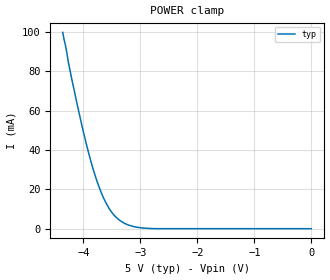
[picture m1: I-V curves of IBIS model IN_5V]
| TEXAS INSTRUMENTS INCORPORATED
| Dual Channel High Speed ESD Protection Device
| Marketing part#   Voltage Range   Package-type   #pins/pkg drawing
| TPD2E1B06DRLR   5.5   SOT   6 / DRL
[IBIS Ver]   4.0
[File name]   tpd2e1b06.ibs
[File Rev]   1.0
[Date]   18-JUL-2013
[Source]
| Texas Instruments Incorporated
| Webench Design Center
| 12500 TI Blvd
| Dallas, TX 75243
| e-mail: elab_scm_ibis@list.ti.com
[Notes]   Revision History:
| Rev 1.0: 18-JUL-2013
| - Initial version of the model
| - Model generated from measurements on Keithley 2420
[Disclaimer]
| This model is designed as an aid for customers of Texas Instruments.
| TI and its licensors and suppliers make no warranties, either expressed
| or implied, with respect to this  model, including the warranties of
| merchantability or fitness for a particular purpose. The model is
| provided solely on an "as is" basis. The entire risk as to its quality
| and performance is with the customer.
[Copyright]
(C) Copyright 2013 Texas Instruments Incorporated. All rights reserved.
|   TPD2E1B06DRL
[Component]   TPD2E1B06DRL
[Manufacturer]   Texas Instruments, Inc.
[Package]   |6 pin DRL SOT package
|   typ   min   max
R_pkg   0.00998   NA   NA
L_pkg   0.60587n   NA   NA
C_pkg   0.18890p   NA   NA
[Pin]   signal_name   model_name   R_pin   L_pin   C_pin
1   IOA1   IN_5V   0.03787   0.61375n   0.10884p
2   IOB1   IN_5V   0.00623   0.52312n   0.18891p
3   NC   NC   0.00998   0.81276n   0.26643p
4   IOB2   GND   0.03772   0.60587n   0.10852p
5   IOA2   GND   0.00623   0.52312n   0.18890p
6   NC   NC   0.00998   0.81270n   0.26639p
| Models and submodels in the file (1): IN_5V (Input)
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|   Model IN_5V
[Model]   IN_5V
Model_type   Input
Vinl = 0
Vinh = 0
|   typ   min   max
C_comp   0.1p   0.1p   0.1p
[Voltage Range]   5   NA   NA
[Temperature Range]   27   NA   NA
[Power Clamp Reference]   5   NA   NA
[GND Clamp Reference]   0   NA   NA
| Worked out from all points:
|   POWER clamp passes 1 mA (typ) near -3.11 V on its own axis
[GND Clamp]
|   Voltage   I(typ)   I(min)   I(max)
-5V       0A         NA         NA
-4.88V    0A         NA         NA
-4.759V   0A         NA         NA
5V        0A         NA         NA
[POWER Clamp]
|   Voltage   I(typ)   I(min)   I(max)
-4.364V   99.78mA    NA         NA
-4.196V   74.73mA    NA         NA
-4.076V   58.72mA    NA         NA
-3.956V   43.78mA    NA         NA
-3.836V   30.86mA    NA         NA
-3.715V   20.41mA    NA         NA
-3.619V   13.96mA    NA         NA
-3.499V   8.161mA    NA         NA
-3.379V   4.596mA    NA         NA
-3.163V   1.418mA    NA         NA
-2.827V   77.93uA    NA         NA
0V        0A         NA         NA
